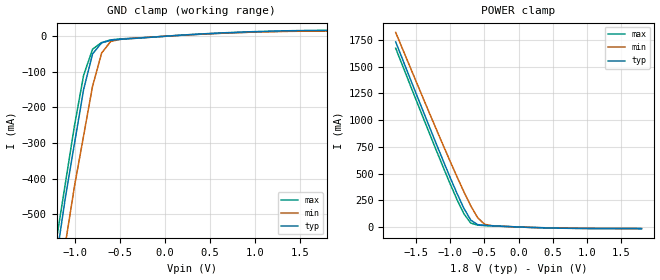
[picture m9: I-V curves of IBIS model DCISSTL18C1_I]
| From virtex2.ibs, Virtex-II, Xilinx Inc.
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|   Model DCISSTL18C1_I
[Model]   DCISSTL18C1_I
Model_type   Input
Vinh = 1.025V
Vinl = 0.775V
Polarity   Non-Inverting
C_comp   10.00pF   10.00pF   10.00pF
[Temperature Range]   25.00   100.00   0.000
[Voltage Range]   1.80V   1.70V   1.90V
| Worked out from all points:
|   GND clamp passes 1 mA (typ) near -0.05 V on its own axis
|   POWER clamp passes 1 mA (typ) near -0.04 V on its own axis
[GND_clamp]
| voltage   I(typ)   I(min)   I(max)
-1.8V     -1.65A     -1.74A     -1.6A
-1.2V     -620mA     -740mA     -570mA
-1.1V     -450mA     -580mA     -410mA
-1V       -300mA     -420mA     -250mA
-900mV    -150mA     -280mA     -110mA
-800mV    -49.55mA   -140mA     -36.2mA
-700mV    -18.49mA   -47.41mA   -17.58mA
-600mV    -11.42mA   -14.71mA   -10.22mA
-500mV    -8.72mA    -8.81mA    -7.55mA
600mV     9.08mA     8.3mA      8.13mA
1.8V      16.63mA    14.79mA    16mA
[POWER_clamp]
| voltage   I(typ)   I(min)   I(max)
-1.8V     1.731A     1.82A      1.672A
-1.4V     1.086A     1.208A     1.026A
-1V       459.3mA    610.7mA    400.1mA
-900mV    311mA      466.7mA    253.6mA
-800mV    173.3mA    327.5mA    122.1mA
-700mV    64.03mA    197.2mA    36.15mA
-600mV    22.11mA    87.38mA    17.53mA
-500mV    15.64mA    25.89mA    13.02mA
-400mV    12.1mA     12.6mA     10.1mA
500mV     -9.974mA   -9.515mA   -8.935mA
1.8V      -15.66mA   -14.79mA   -14.85mA
